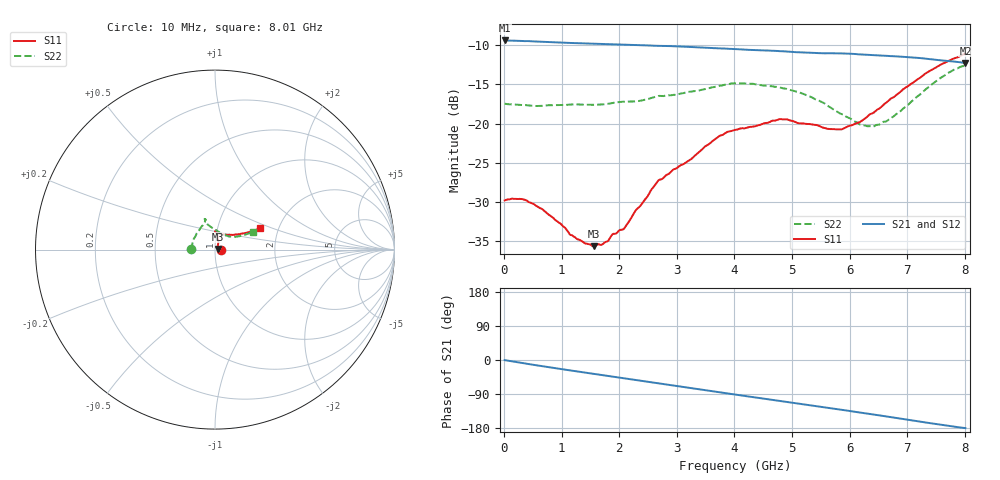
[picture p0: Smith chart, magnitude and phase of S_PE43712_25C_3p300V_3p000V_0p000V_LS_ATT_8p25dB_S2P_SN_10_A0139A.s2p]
! DEVICE ID: PE43712
! File Path: z:\PE43713\PE43713_CHAR_NOM_04292014\AMB\3p300\LS_ATT_8p25dB\PE43713_AMB_3p300V_3p000V_0p000V_LS_ATT_8p25dB_S2P_SN_10_A0139A.s2p
! Serial: 10
! Lot: A0139A
! Temp: 25C
! VDD: 3.300
! VSS: 0.000
! Control_Hi: 3.000
! Control_Lo: 0.000
! Attenuation Step: 8.25dB
! Port 1: RF1
! Port 2: RF2
! ThroughPath:1-2
! IDD: 0.0001466738
! ISS: -1.594e-007
#  Hz  S  RI  R  50
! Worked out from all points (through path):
!   801 points, 10 MHz to 8.01 GHz, reference 50 ohm
!   highest |S21| = -9.41 dB at 10 MHz (marker M1); lowest = -12.3 dB at 8.01 GHz (marker M2)
!   group delay of S21, straight-line fit = 61.8 ps
!   lowest |S11| = -35.6 dB at 1.56 GHz (marker M3), VSWR 1.03, Z = 51.6 + j0.406 ohm
!   |S11| at or under -10 dB: start of sweep to end of sweep
!   |S22| runs from -20.4 to -12.6 dB; largest |S21 - S12| = 0.0012
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1e7  0.0323 0.00011  0.3384 -0.00177  0.3384 -0.00186  -0.1339 0.00084
3e8  0.0328 -0.00386  0.3331 -0.0445  0.333 -0.0445  -0.1304 0.0143
5e8  0.0304 -0.00525  0.3261 -0.0721  0.3261 -0.0721  -0.1279 0.0226
9.6e8  0.0229 -0.00407  0.302 -0.1295  0.3021 -0.1295  -0.1237 0.0438
1.17e9  0.0194 -0.00179  0.2881 -0.1526  0.2882 -0.1528  -0.1208 0.0536
1.35e9  0.0178 0.000199  0.2755 -0.1716  0.2755 -0.1717  -0.1172 0.0608
1.56e9  0.0161 0.00393  0.259 -0.1925  0.2591 -0.1925  -0.1108 0.0711
1.72e9  0.0154 0.00755  0.2456 -0.2074  0.2456 -0.2074  -0.1068 0.0782
2.09e9  0.0142 0.0162  0.2113 -0.2385  0.2113 -0.2383  -0.0988 0.0959
2.68e9  0.0195 0.0388  0.1487 -0.275  0.1487 -0.2751  -0.074 0.1303
3.24e9  0.0157 0.0569  0.0835 -0.2958  0.0836 -0.2958  -0.0616 0.147
3.72e9  0.0136 0.0812  0.0273 -0.3003  0.0271 -0.3002  -0.0558 0.164
4.01e9  0.00994 0.0905  -0.00642 -0.2983  -0.00646 -0.2982  -0.0579 0.171
4.79e9  0.0045 0.1067  -0.0902 -0.2748  -0.0903 -0.275  -0.0526 0.1614
5.35e9  0.0153 0.0974  -0.1419 -0.2443  -0.1418 -0.2442  -0.0414 0.1405
5.63e9  0.0266 0.0885  -0.1648 -0.227  -0.1647 -0.2271  -0.0236 0.1268
5.87e9  0.0384 0.0836  -0.1854 -0.2095  -0.1851 -0.2094  -0.00466 0.1144
6.32e9  0.0759 0.0822  -0.2153 -0.1699  -0.2149 -0.1698  0.0393 0.0877
6.68e9  0.1129 0.0836  -0.2331 -0.1349  -0.2328 -0.135  0.077 0.0729
7.56e9  0.2112 0.1029  -0.2497 -0.0425  -0.2495 -0.0427  0.1734 0.0851
7.81e9  0.2338 0.1134  -0.2476 -0.0187  -0.2475 -0.0188  0.1988 0.0951
8.01e9  0.2503 0.1214  -0.2435 -0.00116  -0.2432 -0.00153  0.211 0.0994
